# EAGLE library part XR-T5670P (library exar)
B8ZS/AMI LINE TRANSCODER
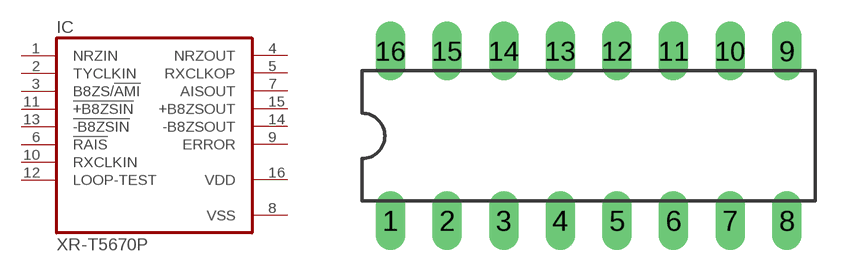
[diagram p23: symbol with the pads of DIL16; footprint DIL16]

Designator prefix IC

## XR-T5670P (OC_FARNELL: unknown; OC_NEWARK: unknown)  [DIL16]
1  NRZIN  in
2  TYCLKIN  in
3  B8ZS/!AMI  in
4  NRZOUT  out
5  RXCLKOP  out
6  !RAIS  in
7  AISOUT  out
8  VSS  pwr
9  ERROR  out
10  RXCLKIN  in
11  !+B8ZSIN  in
12  LOOP-TEST  in
13  !-B8ZSIN  in
14  -B8ZSOUT  out
15  +B8ZSOUT  out
16  VDD  pwr

## Footprint DIL16 (pad centres in mm)
Dual In Line Package
drill 0.813 long: 1 -8.89,-3.81; 2 -6.35,-3.81; 3 -3.81,-3.81; 4 -1.27,-3.81; 5 1.27,-3.81; 6 3.81,-3.81; 7 6.35,-3.81; 8 8.89,-3.81; 9 8.89,3.81; 10 6.35,3.81; 11 3.81,3.81; 12 1.27,3.81; 13 -1.27,3.81; 14 -3.81,3.81; 15 -6.35,3.81; 16 -8.89,3.81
